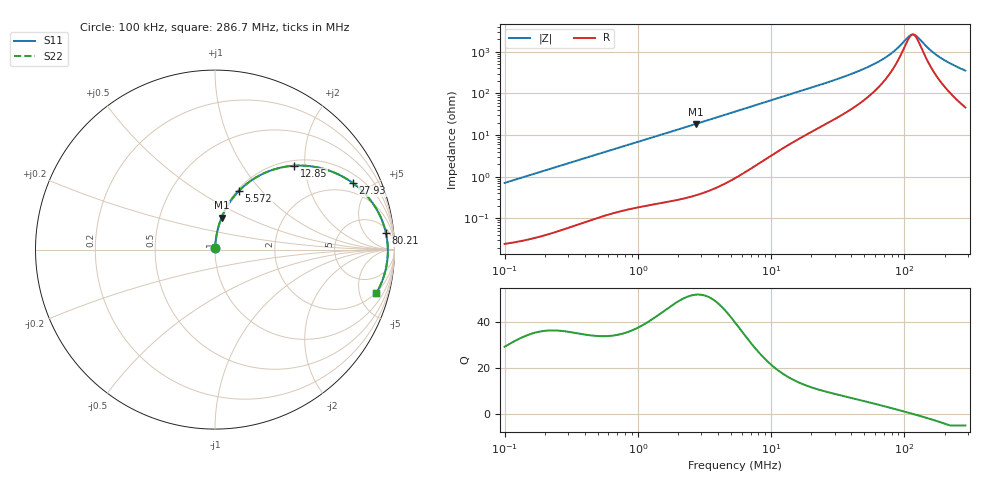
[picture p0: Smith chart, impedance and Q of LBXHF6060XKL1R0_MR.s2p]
! LBXHF6060XKL1R0_MR  S-PARAMETER MODEL  ( General Type )
! Model Generated by TAIYO YUDEN Corporation (http://www.ty-top.com)
! Version 1.0
! TAIYO YUDEN Control No. 220210
! Copyright(c) 2022 TAIYO YUDEN CO.,LTD. All Rights Reserved.
! Product Description (link to TY-COMPAS)
! https://ds.yuden.co.jp/TYCOMPAS/or/detail?pn=LBXHF6060XKL1R0NMR&u=M
! Products Name : Inductors
! Characteristics :
!  Inductance : 1.0 uH , SRF(min) : 80 MHz , DC Resistance(max) : 0.017 Ohm
!  Rated Current : Saturation :7500 mA , Temp Rise : 5800 mA
!  Case Size : 6.0 x 6.0 / 0.236 x 0.236 [mm/inch] , Thickness : 3 / 0.118 [mm/inch]
!  (Conditions: Temperature = 25 degC , DC Bias Current/Voltage = 0A / 0V)
! External Node Assignments :
!  1  o---GGG---o  2
! GND o---------o GND
! Frequency Range : 0.1MHz  -  286.687601MHz  [ 402 STEP ]
# MHz S RI R 50
! Freq[MHz].  S11 Real  S11 Imag  S21 Real  S21 Imag  S12 Real  S12 Imag  S22 Real  S22 Imag
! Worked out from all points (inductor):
!   401 points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, 100 kHz to 286.7 MHz, reference 50 ohm
!   read as one part in series: L = 1.13 uH near 104.1 kHz
!   highest Q = 51.6 at 2.722 MHz (marker M1), where L = 1.08 uH
!   self-resonance near 115.5 MHz
!   S11 on the Smith chart (normalised r, x): 100 kHz: 1.00, +0.01; 5.572 MHz: 1.02, +0.76; 12.85 MHz: 1.11, +1.76; 27.93 MHz: 1.43, +3.88; 80.21 MHz: 8, +17; 286.7 MHz: 1.92, -7.01
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0.1  0.000295 0.00711  0.9997 -0.00711  0.9997 -0.00711  0.000295 0.00711
0.379416  0.00148 0.0266  0.9985 -0.0266  0.9985 -0.0266  0.00148 0.0266
1.439567  0.0118 0.097  0.9882 -0.097  0.9882 -0.097  0.0118 0.097
2.721603  0.0364 0.1779  0.9636 -0.1779  0.9636 -0.1779  0.0364 0.1779
5.354322  0.124 0.3172  0.876 -0.3172  0.876 -0.3172  0.124 0.3172
5.571748  0.1329 0.3267  0.8671 -0.3267  0.8671 -0.3267  0.1329 0.3267
8.29587  0.2523 0.4154  0.7477 -0.4154  0.7477 -0.4154  0.2523 0.4154
12.85344  0.4407 0.4673  0.5593 -0.4673  0.5593 -0.4673  0.4407 0.4673
20.31517  0.6492 0.4353  0.3508 -0.4353  0.3508 -0.4353  0.6492 0.4353
27.93295  0.7682 0.3706  0.2318 -0.3706  0.2318 -0.3706  0.7682 0.3706
50.74841  0.9073 0.2124  0.0927 -0.2124  0.0927 -0.2124  0.9073 0.2124
64.4384  0.9361 0.1483  0.0639 -0.1483  0.0639 -0.1483  0.9361 0.1483
77.07906  0.9502 0.1017  0.0498 -0.1017  0.0498 -0.1017  0.9502 0.1017
80.20907  0.9525 0.0915  0.0475 -0.0915  0.0475 -0.0915  0.9525 0.0915
90.38256  0.9581 0.0613  0.0419 -0.0613  0.0419 -0.0613  0.9581 0.0613
108.1126  0.9625 0.0165  0.0375 -0.0165  0.0375 -0.0165  0.9625 0.0165
117.0713  0.9631 -0.0034  0.0369 0.0034  0.0369 0.0034  0.9631 -0.0034
124.2742  0.9629 -0.0183  0.0371 0.0183  0.0371 0.0183  0.9629 -0.0183
154.6891  0.9581 -0.0737  0.0419 0.0737  0.0419 0.0737  0.9581 -0.0737
181.3877  0.9501 -0.1152  0.0499 0.1152  0.0499 0.1152  0.9501 -0.1152
225.7806  0.9315 -0.1748  0.0685 0.1748  0.0685 0.1748  0.9315 -0.1748
286.6876  0.8988 -0.243  0.1012 0.243  0.1012 0.243  0.8988 -0.243
